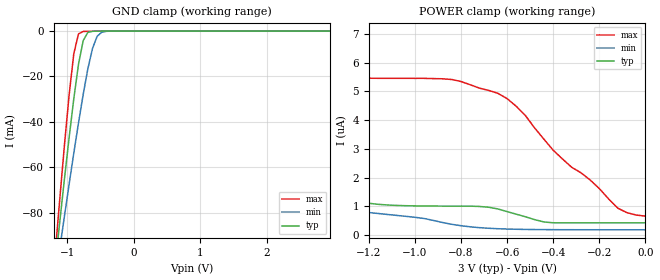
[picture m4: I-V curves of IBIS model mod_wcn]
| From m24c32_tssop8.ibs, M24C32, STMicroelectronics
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|   Model mod_wcn
[Model]   mod_wcn
Model_type Input
Vinl   =   0.900V
Vinh   =   2.100V
C_comp   2.219pF   2.024pF   2.433pF
[Temperature Range]  25.0000   0.1250k   -40.0000
[Voltage Range]   3.0000V   1.8000V   5.5000V
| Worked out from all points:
|   GND clamp passes 1 mA (typ) near -0.70 V on its own axis
[GND_clamp]
|Voltage   I(typ)   I(min)   I(max)
-3V       -632.3mA   -502.5mA   -782.2mA
-1.18V    -103mA     -110.1mA   -98.29mA
-1.11V    -83.81mA   -95.65mA   -73.75mA
-1.04V    -65mA      -81.41mA   -50.05mA
-970mV    -46.82mA   -67.4mA    -28mA
-900mV    -29.7mA    -53.72mA   -9.899mA
-830mV    -14.69mA   -40.49mA   -1.245mA
-760mV    -4.25mA    -28mA      -159.3uA
-620mV    -83.69uA   -7.672mA   -65.52uA
-550mV    -26.12uA   -2.289mA   -45.81uA
-480mV    -12.79uA   -464.3uA   -27.85uA
2.95V     1.011uA    747.3nA    5.256uA
[POWER_clamp]
|Voltage   I(typ)   I(min)   I(max)
-3V       5.116uA    3.317uA    27.04uA
-2.8V     4.752uA    2.691uA    21.35uA
-1.76V    2.963uA    1.34uA     7.424uA
-1.72V    2.893uA    1.296uA    7.028uA
-1.6V     2.648uA    1.168uA    6.154uA
-1.44V    1.75uA     1.008uA    5.597uA
-1.2V     1.11uA     789.3nA    5.456uA
-800mV    1.011uA    330.8nA    5.342uA
-600mV    820.9nA    215.5nA    4.746uA
-440mV    461nA      195.8nA    3.333uA
-120mV    432.1nA    190.6nA    941.2nA
0V        432.1nA    190.4nA    664.3nA
